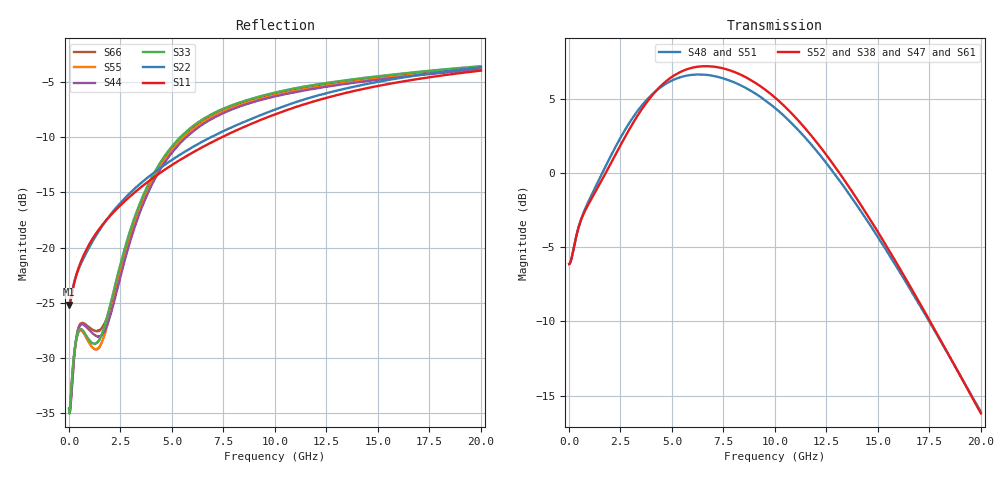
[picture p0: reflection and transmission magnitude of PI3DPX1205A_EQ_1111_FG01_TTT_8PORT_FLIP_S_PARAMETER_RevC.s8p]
! NPort=8 DATA=2000 NOISE=0 GROUPDELAY=0 COMPLEX_DATAFORMAT=POLAR
! NumOfBlock=1 NumOfParam=0
! .MODEL Smodel S TSTONEFILE=PI3DPX1205A_EQ_1111_FG01_TTT_8PORT_FLIP_S_PARAMETER_RevC.s8p TYPE=S
!  -- The above .MODEL line can be used for the S element in the netlist.
! The s parameter is extracted from the linear redriver, it is not bi-directional;
! only s(5,1)s(6,2)s(3,7)s(4,8) should be the insertion loss
!  Port definition:
!  Port1 = AIP
!  Port2 = AIN
!  Port3 = BOP
!  Port4 = BON
!  Port5 = AOP
!  Port6 = AON
!  Port7 = BIP
!  Port8 = BIN
# Hz S MA R  50
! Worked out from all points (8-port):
!   2000 points, 10 MHz to 20 GHz, reference 50 ohm
!   strongest paths, dB at 10 MHz, 5.01 GHz, 10.01 GHz, 15.01 GHz, 20 GHz:
!     S52: -6.1, 6.5, 5.1, -4.0, -16.2
!     S38: -6.1, 6.5, 5.1, -4.0, -16.2
!     S47: -6.1, 6.5, 5.1, -4.0, -16.1
!     S61: -6.1, 6.5, 5.1, -4.0, -16.1
!     S48: -6.1, 6.2, 4.4, -4.3, -16.1
!     S51: -6.1, 6.2, 4.4, -4.3, -16.1
!   lowest |S11| = -25.2 dB at 10 MHz (marker M1), VSWR 1.12, Z = 44.8 - j0.115 ohm
!   |S11| at or under -10 dB: start of sweep to 7.443 GHz
